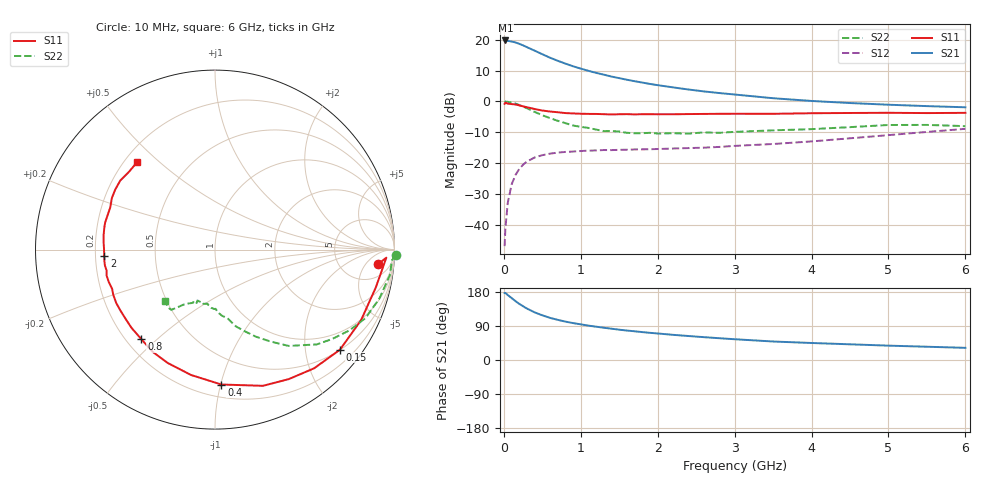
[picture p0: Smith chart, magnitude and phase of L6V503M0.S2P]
!  INFINEON TECHNOLOGIES Small Signal Semiconductors
! BFR380L3 , Si-NPN RF-Transistor in TSLP-3-1
!  Vce=0.5 V,  Ic=3 mA
! Common Emitter S-Parameters:  07. March 2005
#  GHz  S  MA  R  50
! f  S11  S21  S12  S22
! GHz  Mag  Ang  Mag  Ang  Mag  Ang  Mag  Ang
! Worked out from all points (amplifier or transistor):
!   36 points, 10 MHz to 6 GHz, reference 50 ohm
!   highest |S21| = 19.7 dB at 20 MHz (marker M1)
!   |S21| within 3 dB of that: start of sweep to 373.3 MHz
!   unconditionally stable (mu >= 1): 2.399 GHz to 5.155 GHz
!   at 250 MHz: K = 0.13, MSG = 19.3 dB, |S12| = -20.5 dB
!   at 1.4 GHz: K = 0.68, MSG = 11.9 dB, |S12| = -15.8 dB
!   at 6 GHz: K = 0.98, MSG = 3.5 dB, |S12| = -8.9 dB
!   S11 on the Smith chart (normalised r, x): 10 MHz: 11, -11; 150 MHz: 0.51, -2.77; 400 MHz: 0.29, -1.01; 800 MHz: 0.26, -0.45; 2 GHz: 0.24, -0.03; 6 GHz: 0.25, +0.42
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0.01  0.9124 -5.1  9.664 176.7  0.0045 82.5  1.011 -1.7
0.02  0.9556 -2.7  9.715 177.0  0.0087 87.9  0.9879 -3.4
0.05  0.9203 -13.3  9.601 171.6  0.0223 83.0  0.9841 -8.4
0.1  0.9038 -25.8  9.336 163.6  0.0447 76.7  0.9559 -16.5
0.15  0.892 -38.7  9.03 155.6  0.0637 68.9  0.9216 -24.4
0.2  0.8617 -50.1  8.567 148.2  0.0801 63.5  0.8756 -30.8
0.25  0.8305 -60.3  8.087 141.9  0.0942 57.9  0.8207 -37.4
0.3  0.8046 -70.6  7.569 135.7  0.106 53.6  0.7746 -43.0
0.4  0.7525 -87.3  6.642 125.7  0.1232 46.3  0.6756 -52.6
0.5  0.7113 -100.8  5.812 117.9  0.1342 41.1  0.5968 -59.0
0.6  0.6845 -112.6  5.105 111.2  0.1423 37.0  0.5357 -64.9
0.8  0.646 -129.4  4.095 101.3  0.1516 32.6  0.444 -74.7
0.9  0.6376 -136.9  3.705 97.4  0.1539 31.2  0.4064 -78.0
1.1  0.6269 -147.1  3.127 90.7  0.1591 29.7  0.3711 -83.9
1.5  0.6188 -163.1  2.38 80.0  0.164 29.6  0.3247 -93.8
2  0.6182 -176.5  1.832 70.0  0.169 32.5  0.3012 -104.0
2.2  0.6183 179.6  1.686 66.4  0.1722 33.9  0.3043 -104.3
2.8  0.6288 168.6  1.365 57.5  0.1827 40.0  0.3092 -112.6
3.5  0.6289 158.3  1.125 48.8  0.2038 45.6  0.3393 -117.4
4.5  0.6485 149.1  0.94 41.4  0.2521 53.2  0.3824 -122.9
5.5  0.6462 138.2  0.838 35.0  0.3197 55.5  0.4155 -129.4
6  0.6519 131.8  0.802 32.1  0.3588 55.0  0.3969 -134.2
